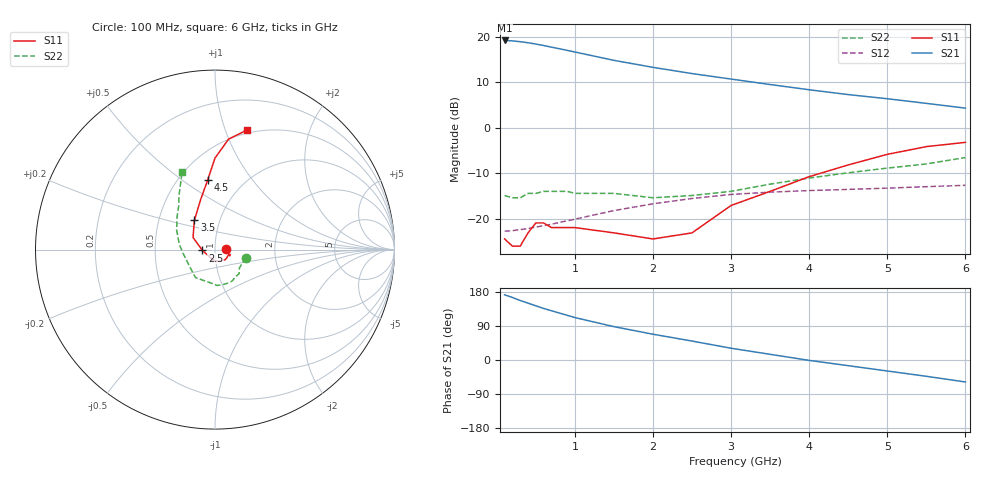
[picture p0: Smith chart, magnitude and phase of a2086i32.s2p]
!  MSA-2086 S AND NOISE PARAMETERS
!  Id = 32 mA  LAST UPDATED 06-27-94
# ghz s ma r 50
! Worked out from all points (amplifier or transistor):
!   20 points, 100 MHz to 6 GHz, reference 50 ohm
!   highest |S21| = 19.2 dB at 100 MHz (marker M1)
!   |S21| within 3 dB of that: start of sweep to 1.126 GHz
!   unconditionally stable (mu >= 1): start of sweep to 4.933 GHz
!   at 400 MHz: K = 1.06, MAG = 18.9 dB, |S12| = -22.2 dB
!   at 1.5 GHz: K = 1.04, MAG = 15.3 dB, |S12| = -18.2 dB
!   at 6 GHz: K = 0.74, MSG = 8.5 dB, |S12| = -12.7 dB
!   S11 on the Smith chart (normalised r, x): 100 MHz: 1.13, +0.00; 2.5 GHz: 0.87, -0.01; 3.5 GHz: 0.76, +0.26; 4.5 GHz: 0.69, +0.63; 6 GHz: 0.47, +1.19
0.1  0.06 1.0  9.08 172.0  0.073 4.0  0.18 -15.0
0.2  0.05 -5.0  8.98 165.0  0.074 7.0  0.17 -26.0
0.3  0.05 -10.0  8.8 157.0  0.076 10.0  0.17 -37.0
0.4  0.07 -15.0  8.57 150.0  0.078 13.0  0.19 -45.0
0.5  0.09 -18.0  8.29 143.0  0.081 15.0  0.19 -53.0
0.6  0.09 -22.0  7.99 136.0  0.084 18.0  0.2 -62.0
0.7  0.08 -23.0  7.66 130.0  0.087 20.0  0.2 -71.0
0.8  0.08 -31.0  7.37 124.0  0.091 21.0  0.2 -80.0
0.9  0.08 -34.0  7.07 118.0  0.095 23.0  0.2 -87.0
1  0.08 -44.0  6.78 112.0  0.099 23.0  0.19 -94.0
1.5  0.07 -71.0  5.49 88.0  0.123 24.0  0.19 -125.0
2  0.06 -99.0  4.6 68.0  0.146 22.0  0.17 -145.0
2.5  0.07 -176.0  3.93 50.0  0.167 17.0  0.18 -174.0
3  0.14 151.0  3.42 31.0  0.185 10.0  0.2 172.0
3.5  0.2 125.0  2.98 15.0  0.196 3.0  0.24 153.0
4  0.29 106.0  2.61 -1.0  0.204 -3.0  0.28 139.0
4.5  0.39 96.0  2.31 -15.0  0.21 -8.0  0.32 129.0
5  0.51 90.0  2.08 -29.0  0.217 -12.0  0.36 124.0
5.5  0.62 83.0  1.85 -43.0  0.225 -16.0  0.4 119.0
6  0.69 75.0  1.64 -58.0  0.233 -22.0  0.47 113.0
